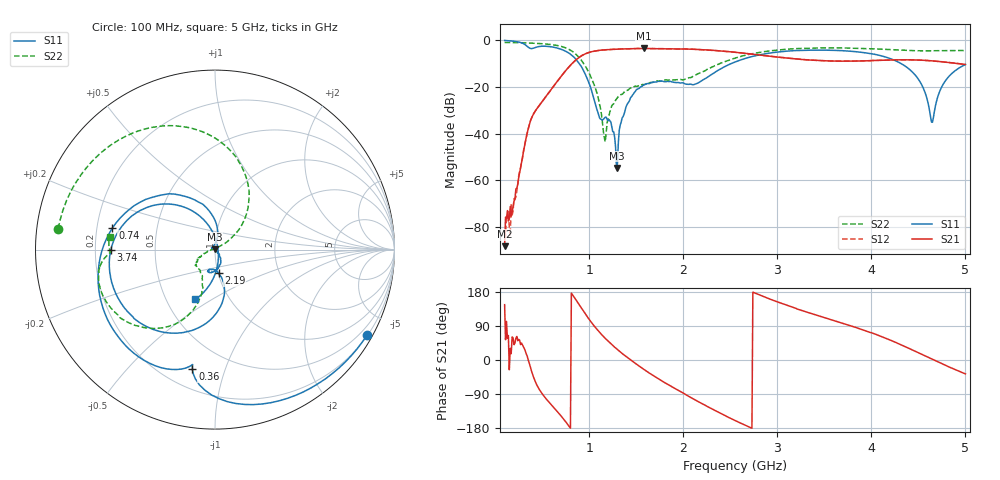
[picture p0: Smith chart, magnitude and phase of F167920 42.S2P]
!  2-Port S-parameters saved by WinCal
! VAR MeasName=S-Parameters (CALIBRATED_DATA) read from VNA (N5242A)
! VAR MeasDate=2016-11-22 9:57:33
! VAR NAME=F167920 42
! VAR FILENAME=F167920 42.S2P
! VAR DATE=2016-11-22 9:57:33
! VAR PHYS_PORTS=1,2
# Hz S DB R 50
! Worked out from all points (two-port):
!   491 points, 100 MHz to 5 GHz, reference 50 ohm
!   highest |S21| = -3.66 dB at 1.58 GHz (marker M1); lowest = -88.0 dB at 100 MHz (marker M2)
!   |S21| within 3 dB of the highest: 922.9 MHz to 2.855 GHz (1.932 GHz wide, 102 % of centre)
!   lowest |S11| = -54.7 dB at 1.29 GHz (marker M3), VSWR 1.00, Z = 50 + j0.18 ohm
!   |S11| at or under -10 dB: 891.7 MHz to 2.516 GHz (1.624 GHz wide, 95.3 % of centre); 4.311 GHz to end of sweep
!   |S22| runs from -43.5 to -1.1 dB; largest |S21 - S12| = 0.0014
!   S11 on the Smith chart (normalised r, x): 100 MHz: 0.22, -3.82; 360 MHz: 0.32, -0.78; 740 MHz: 0.26, +0.10; 2.19 GHz: 1.00, -0.27; 3.74 GHz: 0.27, -0.00; 5 GHz: 0.70, -0.42
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1e8  -0.25 -29.3  -88.03 146.0  -83.12 60.5  -1.10 172.4
1.7e8  -0.47 -49.4  -75.21 16.5  -69.93 49.8  -1.15 167.0
3.6e8  -3.37 -100.7  -36.46 -6.5  -36.51 -6.8  -1.35 151.3
5.2e8  -2.69 -127.9  -25.20 -95.8  -25.24 -95.7  -1.70 134.9
7.4e8  -4.67 168.2  -13.59 -159.9  -13.58 -159.9  -3.27 100.5
9.2e8  -11.64 105.0  -6.73 136.1  -6.73 136.1  -8.93 57.7
1.07e9  -28.11 85.7  -4.70 84.5  -4.71 84.5  -21.17 33.6
1.16e9  -33.44 151.4  -4.27 59.6  -4.26 59.6  -41.72 85.3
1.24e9  -37.16 144.4  -4.06 40.8  -4.06 40.7  -28.05 -166.2
1.29e9  -54.68 103.1  -3.98 29.7  -3.97 29.7  -25.24 -161.5
1.4e9  -27.77 -53.0  -3.82 7.7  -3.82 7.7  -21.59 -156.1
1.58e9  -19.23 -82.7  -3.66 -24.5  -3.66 -24.5  -19.11 -150.6
1.74e9  -17.67 -100.7  -3.75 -50.1  -3.75 -50.1  -17.55 -144.4
2.19e9  -17.58 -81.5  -4.19 -114.0  -4.19 -114.0  -13.85 -110.5
2.55e9  -9.45 -86.7  -5.28 -159.5  -5.27 -159.5  -7.79 -113.0
3.37e9  -4.38 -152.7  -8.67 121.9  -8.65 121.9  -3.51 -152.1
3.74e9  -4.72 -179.9  -9.09 93.5  -9.07 93.5  -3.48 -165.1
4.19e9  -7.83 141.9  -8.59 53.6  -8.61 53.6  -4.17 -175.5
4.49e9  -16.22 107.4  -8.59 20.3  -8.61 20.4  -4.65 -178.3
4.65e9  -35.15 -8.3  -8.96 1.6  -8.97 1.7  -4.66 -179.5
4.77e9  -18.49 -86.9  -9.41 -12.1  -9.41 -12.0  -4.60 178.8
5e9  -10.53 -111.5  -10.50 -36.7  -10.48 -36.6  -4.57 173.3
